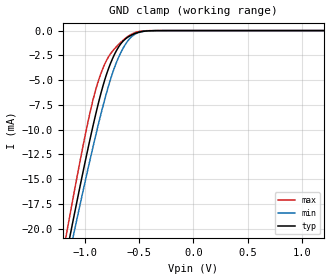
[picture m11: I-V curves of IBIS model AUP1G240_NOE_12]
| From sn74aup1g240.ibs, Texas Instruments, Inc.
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[Model]   AUP1G240_NOE_12
Model_type  Input
Vinl=0.420
Vinh=0.715
| variable   typ   min   max
C_comp   1.69pF   1.48pF   1.91pF
[Temperature Range]   40   100   -40
| Ambient temperature   25   85   -40
[Voltage range]   1.2   1.1   1.3
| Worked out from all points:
|   GND clamp passes 1 mA (typ) near -0.64 V on its own axis
[GND Clamp]
| AUP1G240_NOE_12
|   Voltage   I(typ)   I(min)   I(max)
-3.6V     -171.6mA   -163.5mA   -181.1mA
-1.18V    -23.34mA   -24.74mA   -21.39mA
-1.155V   -21.94mA   -23.43mA   -19.88mA
-1.13V    -20.55mA   -22.13mA   -18.38mA
-1.11V    -19.45mA   -21.09mA   -17.19mA
-1.09V    -18.36mA   -20.06mA   -16.01mA
-950mV    -11mA      -13.08mA   -8.304mA
-850mV    -6.372mA   -8.471mA   -4.359mA
-715mV    -2.201mA   -3.455mA   -1.73mA
-560mV    -408.6uA   -549.1uA   -322.3uA
-345mV    -4.45uA    -6.672uA   -797.7nA
1.2V      66.99pA    417.3pA    12.63pA
